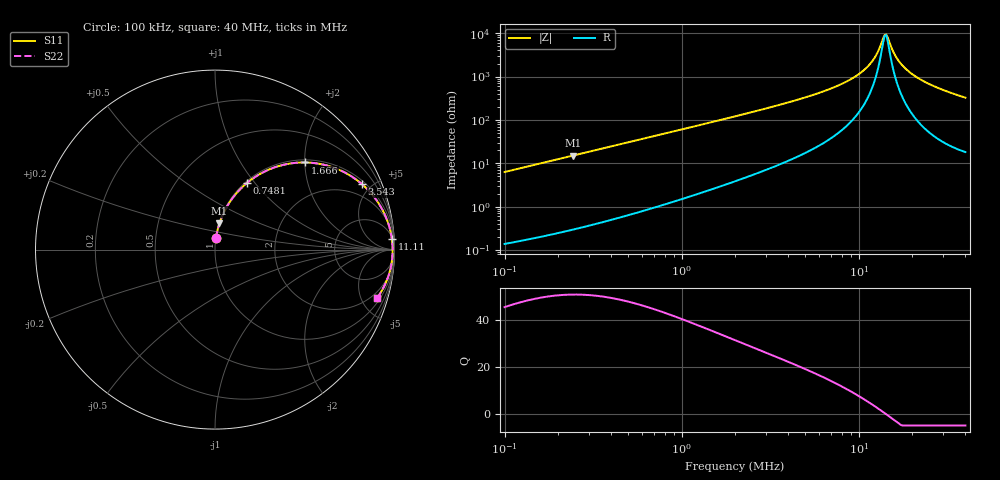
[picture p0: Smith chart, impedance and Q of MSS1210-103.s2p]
# MHz S MA R 50
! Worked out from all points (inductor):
!   263 points, 100 kHz to 40 MHz, reference 50 ohm
!   read as one part in series: L = 9.95 uH near 102.3 kHz
!   highest Q = 50.9 at 244 kHz (marker M1), where L = 9.82 uH
!   self-resonance near 13.97 MHz
!   S11 on the Smith chart (normalised r, x): 100 kHz: 1.00, +0.13; 748.1 kHz: 1.02, +0.90; 1.666 MHz: 1.06, +2.00; 3.543 MHz: 1.19, +4.41; 11.11 MHz: 7, +32; 40 MHz: 1.36, -6.51
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0.1  0.06264 85.2  0.9967 -3.6  0.9967 -3.6  0.06264 85.2
0.2439661  0.1485 80.3  0.986 -8.5  0.986 -8.5  0.1485 80.3
0.2735188  0.1656 79.3  0.9829 -9.5  0.9829 -9.5  0.1656 79.3
0.473526  0.2758 72.8  0.9555 -16.0  0.9555 -16.0  0.2758 72.8
0.7481253  0.4088 64.6  0.9034 -24.1  0.9034 -24.1  0.4088 64.6
1.665627  0.6976 44.1  0.6962 -44.2  0.6962 -44.2  0.6976 44.1
2  0.7581 38.9  0.6285 -49.3  0.6285 -49.3  0.7581 38.9
3.542568  0.8969 23.9  0.4062 -63.7  0.4062 -63.7  0.8969 23.9
5.470376  0.9525 14.8  0.2557 -72.0  0.2557 -72.0  0.9525 14.8
8.447266  0.9795 7.4  0.1302 -77.2  0.1302 -77.2  0.9795 7.4
9.913725  0.9847 5.1  0.08888 -77.6  0.08888 -77.6  0.9847 5.1
11.11462  0.9872 3.4  0.06049 -76.1  0.06049 -76.1  0.9872 3.4
12.46098  0.9889 1.8  0.0331 -69.4  0.0331 -69.4  0.9889 1.8
13.04413  0.9893 1.2  0.02276 -61.3  0.02276 -61.3  0.9893 1.2
13.97043  0.9896 0.2  0.01095 -18.1  0.01095 -18.1  0.9896 0.2
14.29359  0.9896 -0.1  0.01058 11.5  0.01058 11.5  0.9896 -0.1
14.96251  0.9896 -0.8  0.01682 51.5  0.01682 51.5  0.9896 -0.8
15.66273  0.9895 -1.4  0.02656 65.9  0.02656 65.9  0.9895 -1.4
16.77498  0.9889 -2.4  0.04265 73.8  0.04265 73.8  0.9889 -2.4
20.14254  0.9858 -5.0  0.08813 78.2  0.08813 78.2  0.9858 -5.0
26.50285  0.9755 -9.3  0.1618 76.7  0.1618 76.7  0.9755 -9.3
40  0.9415 -16.8  0.2888 70.1  0.2888 70.1  0.9415 -16.8
